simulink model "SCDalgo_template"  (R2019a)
settings: configuration reference "configurationSettings" (kept in a data dictionary, not in this file)
undefined symbols (not defined in the file or in its folder): SCDalgo_template_fp, SCDalgo_template_tp

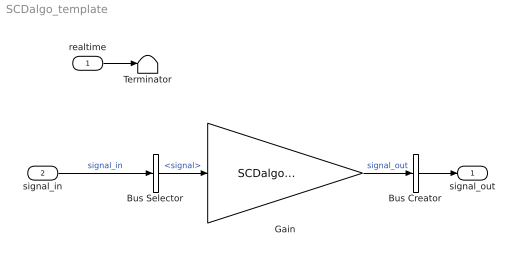
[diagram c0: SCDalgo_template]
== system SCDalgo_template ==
  realtime : Inport  OutDataTypeStr=single  PortDimensions=1  SampleTime=SCDalgo_template_fp.timing.dt  Interpolate=off
  signal_in : Inport  Port=2  OutDataTypeStr=Bus: SCDalgo_template_inBus  PortDimensions=1  SampleTime=SCDalgo_template_fp.timing.dt  Interpolate=off
  Bus Creator : BusCreator  Inputs=1  OutDataTypeStr=Bus: SCDalgo_template_outBus
  Bus Selector : BusSelector  OutputSignals=signal
  Gain : Gain  Gain=SCDalgo_template_tp.gain
  Terminator : Terminator
  signal_out : Outport  OutDataTypeStr=Bus: SCDalgo_template_outBus
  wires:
  signal_in/1 -> Bus Selector/1  "signal_in"
  Bus Selector/1 -> Gain/1  "<signal>"
  Gain/1 -> Bus Creator/1  "signal_out"
  Bus Creator/1 -> signal_out/1
  realtime/1 -> Terminator/1
